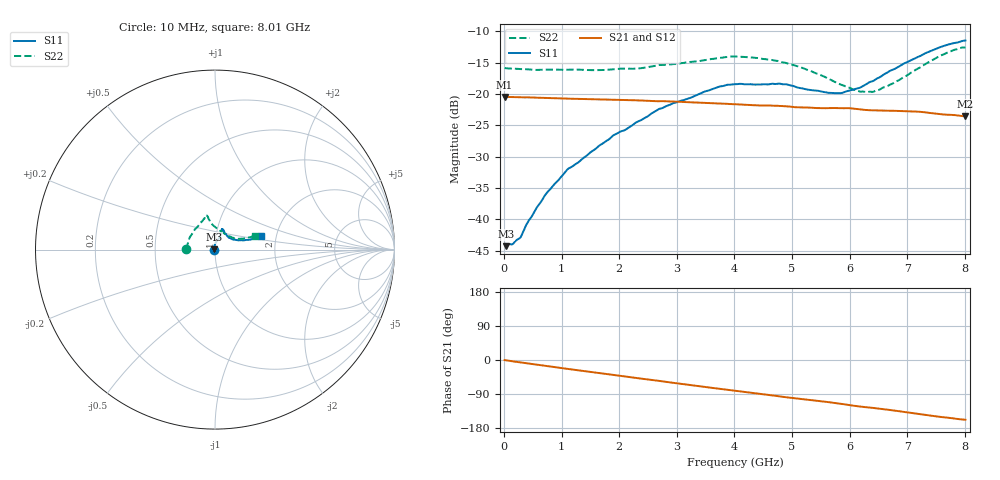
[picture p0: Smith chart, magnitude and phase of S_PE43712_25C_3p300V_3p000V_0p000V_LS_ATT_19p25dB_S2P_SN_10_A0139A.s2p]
! DEVICE ID: PE43712
! File Path: z:\PE43713\PE43713_CHAR_NOM_04292014\AMB\3p300\LS_ATT_19p25dB\PE43713_AMB_3p300V_3p000V_0p000V_LS_ATT_19p25dB_S2P_SN_10_A0139A.s2p
! Serial: 10
! Lot: A0139A
! Temp: 25C
! VDD: 3.300
! VSS: 0.000
! Control_Hi: 3.000
! Control_Lo: 0.000
! Attenuation Step: 19.25dB
! Port 1: RF1
! Port 2: RF2
! ThroughPath:1-2
! IDD: 0.000146803
! ISS: -2.192e-007
#  Hz  S  RI  R  50
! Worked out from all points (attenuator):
!   801 points, 10 MHz to 8.01 GHz, reference 50 ohm
!   highest |S21| = -20.48 dB at 10 MHz (marker M1); lowest = -23.6 dB at 8 GHz (marker M2)
!   lowest |S11| = -44.3 dB at 30 MHz (marker M3), VSWR 1.01, Z = 49.4 + j0.136 ohm
!   |S11| at or under -10 dB: start of sweep to end of sweep
!   |S22| runs from -19.7 to -12.6 dB; largest |S21 - S12| = 0.00033
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1e7  -0.00635 0.000554  0.0946 -0.000471  0.0946 -0.000459  -0.1606 0.0011
3e7  -0.00595 0.00138  0.0945 -0.00121  0.0946 -0.00121  -0.16 0.00286
1.5e8  -0.00513 0.00374  0.0941 -0.00564  0.0942 -0.00565  -0.1585 0.0106
2.7e8  -0.00443 0.00548  0.0935 -0.00994  0.0935 -0.00998  -0.1569 0.0169
4.2e8  -0.00408 0.00868  0.0926 -0.0152  0.0925 -0.0153  -0.1548 0.0249
7.4e8  -0.00377 0.0157  0.0891 -0.0257  0.0892 -0.0257  -0.1498 0.0438
1.1e9  -0.00237 0.0249  0.084 -0.0365  0.0841 -0.0365  -0.1422 0.0636
1.35e9  5.63e-05 0.0301  0.0801 -0.0434  0.0801 -0.0434  -0.1358 0.0756
1.91e9  0.00875 0.0462  0.0691 -0.0572  0.0691 -0.0572  -0.1161 0.1065
2.34e9  0.018 0.0578  0.059 -0.0662  0.059 -0.0662  -0.0978 0.1261
2.68e9  0.0268 0.0705  0.0503 -0.0715  0.0502 -0.0715  -0.0823 0.1482
3.71e9  0.0389 0.1062  0.0211 -0.081  0.0211 -0.0811  -0.0545 0.1845
4.01e9  0.0401 0.1126  0.0126 -0.0818  0.0126 -0.0818  -0.053 0.1914
4.76e9  0.0438 0.1124  -0.00769 -0.0798  -0.00762 -0.0799  -0.0381 0.1786
5.35e9  0.0562 0.0909  -0.0218 -0.0744  -0.0218 -0.0743  -0.0233 0.1486
5.82e9  0.0738 0.0691  -0.0326 -0.0696  -0.0326 -0.0697  0.00814 0.1196
6.18e9  0.0961 0.0575  -0.0408 -0.063  -0.0407 -0.0631  0.0418 0.0954
6.4e9  0.1137 0.0547  -0.0438 -0.0595  -0.0437 -0.0595  0.0648 0.0809
6.68e9  0.1414 0.052  -0.0486 -0.0548  -0.0486 -0.0549  0.0961 0.0667
7.55e9  0.2252 0.0623  -0.0596 -0.0348  -0.0595 -0.0348  0.1868 0.0672
8e9  0.255 0.0755  -0.061 -0.0252  -0.061 -0.0253  0.2212 0.0769
8.01e9  0.2555 0.0762  -0.0611 -0.0251  -0.061 -0.0252  0.2217 0.0769
